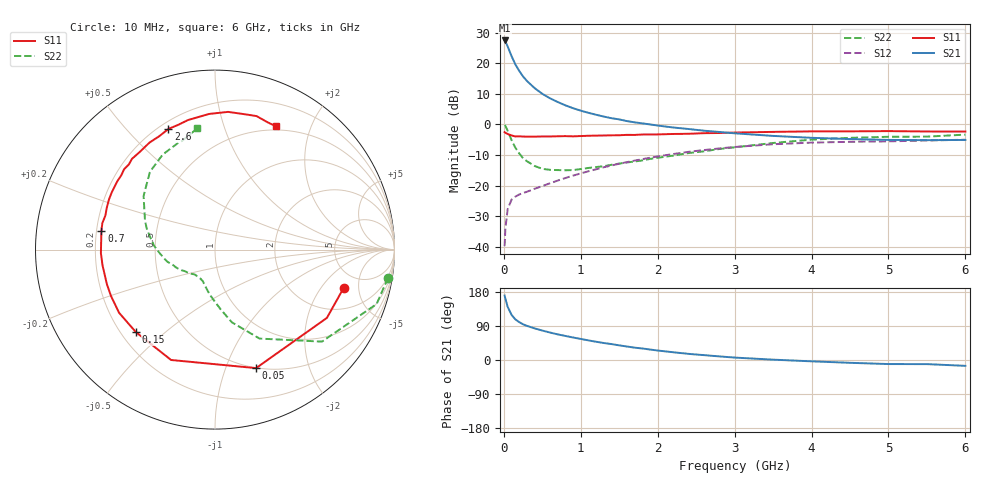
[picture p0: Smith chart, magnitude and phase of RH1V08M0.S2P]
! SIEMENS Small Signal Semiconductors
! BFR106
! Si NPN RF Bipolar Junction Transistor in SOT23
! VCE = 1 V  IC = 8 mA
! Common Emitter S-Parameters:  August  1996
# GHz  S  MA  R  50
!  f  S11  S21  S12  S22
! GHz  MAG  ANG  MAG  ANG  MAG  ANG  MAG  ANG
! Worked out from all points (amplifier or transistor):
!   36 points, 10 MHz to 6 GHz, reference 50 ohm
!   highest |S21| = 27.5 dB at 10 MHz (marker M1)
!   |S21| within 3 dB of that: start of sweep to 66.26 MHz
!   unconditionally stable (mu >= 1): 495.2 MHz to 2.965 GHz; 3.674 GHz to end of sweep
!   at 250 MHz: K = 0.66, MSG = 19.1 dB, |S12| = -22.4 dB
!   at 1.4 GHz: K = 1.14, MAG = 5.5 dB, |S12| = -13.4 dB
!   at 6 GHz: K = 1.03, MAG = -1.1 dB, |S12| = -5.0 dB
!   S11 on the Smith chart (normalised r, x): 10 MHz: 3.54, -3.40; 50 MHz: 0.50, -1.28; 150 MHz: 0.26, -0.40; 700 MHz: 0.22, +0.08; 2.6 GHz: 0.24, +0.66; 6 GHz: 0.46, +1.51
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0.01  0.7485 -16.4  23.7 170.1  0.0102 84.4  0.9768 -9.3
0.02  0.7304 -31.4  22.91 162.1  0.0198 74.6  0.9502 -18.6
0.05  0.6988 -70.9  18.86 140.2  0.0413 57.6  0.7862 -40.7
0.1  0.6619 -111.7  13.17 119.2  0.0587 43.8  0.5544 -63.4
0.15  0.6369 -133.8  9.599 107.1  0.066 38.6  0.4161 -76.9
0.2  0.64 -146.6  7.523 99.9  0.0715 37.8  0.3351 -84.5
0.25  0.6345 -155.9  6.104 94.2  0.0757 38.3  0.2805 -91.6
0.3  0.6324 -162.2  5.154 90.1  0.0792 39.6  0.2505 -97.0
0.4  0.6327 -171.9  3.935 83.4  0.0887 43.0  0.2094 -105.3
0.5  0.6361 -178.2  3.175 77.7  0.0982 45.8  0.1881 -111.3
0.6  0.636 175.6  2.681 72.5  0.1091 48.2  0.1809 -116.6
0.7  0.6414 170.7  2.332 67.6  0.1208 50.3  0.1794 -121.8
0.9  0.6396 162.7  1.846 59.4  0.1456 52.4  0.1795 -130.0
1.1  0.6534 154.7  1.552 51.7  0.1714 53.4  0.1946 -137.3
1.3  0.6603 147.9  1.346 44.8  0.1996 53.0  0.2079 -145.0
1.6  0.6761 138.5  1.136 35.6  0.2421 51.3  0.2388 -155.5
2.2  0.699 121.5  0.893 20.5  0.3282 44.3  0.3089 -176.3
2.6  0.7205 111.1  0.791 12.9  0.3812 38.2  0.3636 170.0
3.5  0.7565 92.5  0.65 0.9  0.4748 23.1  0.4976 143.1
4.5  0.7717 78.1  0.577 -7.4  0.5203 7.4  0.6044 118.8
5.5  0.7675 67.6  0.554 -10.9  0.5467 -2.0  0.6323 106.9
6  0.766 63.7  0.558 -15.4  0.5631 -8.6  0.6822 98.4
